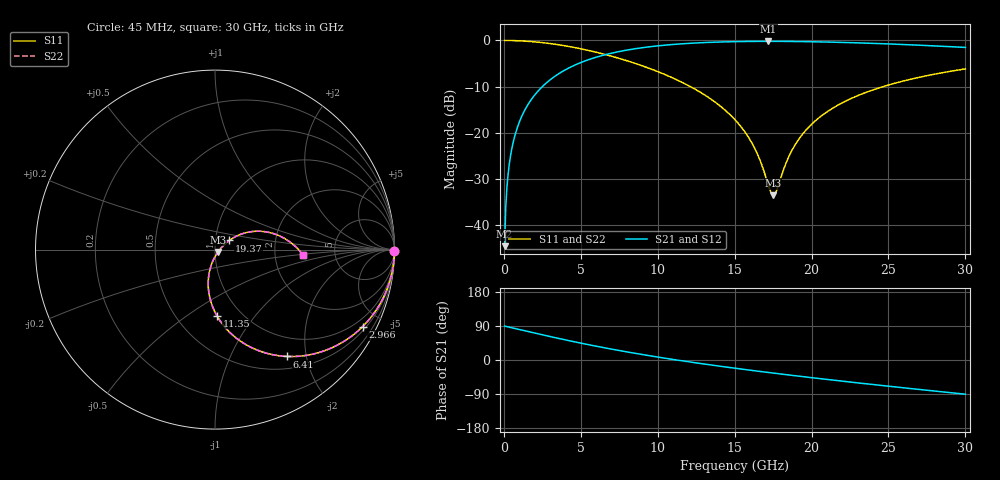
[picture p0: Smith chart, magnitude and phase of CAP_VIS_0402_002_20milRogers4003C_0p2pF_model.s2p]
! S-parameter model data by Modelithics Inc.  support@modelithics.com  813-866-6335  Tampa FL USA
! S-Parameter data specifications:
! Substrate: 20-mil Rogers 4003C, substrate thickness, H=0.508mm, Dielectric constant, Er=3.75
! PCB Mounting Pad Footprint: Pad width, PadW=0.50mm , Pad length, PadL=0.50mm , Pad gap, PadG (edge-to-edge)=0.40mm , Reference planes=1.4mm apart
! Created Wed Nov 18 12:41:56 2015
# hz S ma R 50
! 2 Port Network Data from SP1.SP block
! freq  magS11  angS11  magS21  angS21  magS12  angS12  magS22  angS22
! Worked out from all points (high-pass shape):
!   401 points, 45 MHz to 30 GHz, reference 50 ohm
!   highest |S21| = -0.19 dB at 17.19 GHz (marker M1); lowest = -44.5 dB at 45 MHz (marker M2)
!   |S21| within 3 dB of the highest: 6.465 GHz to end of sweep
!   lowest |S11| = -33.5 dB at 17.49 GHz (marker M3), VSWR 1.04, Z = 51.7 - j1.36 ohm
!   |S11| at or under -10 dB: 12.13 GHz to 24.65 GHz (12.52 GHz wide, 68.1 % of centre)
!   |S22| runs from -33.5 to 0.0 dB; largest |S21 - S12| = 0
!   S11 on the Smith chart (normalised r, x): 45 MHz: open; 2.966 GHz: 0.65, -3.97; 6.41 GHz: 0.68, -1.66; 11.35 GHz: 0.78, -0.66; 19.37 GHz: 1.17, +0.12; 30 GHz: 2.92, -0.24
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4.5e7  1 -0.4  0.00593 89.5  0.00593 89.5  1 -0.4
3.4455e8  0.9989 -3.3  0.04525 86.6  0.04525 86.6  0.9989 -3.3
5.692125e8  0.9971 -5.4  0.07461 84.5  0.07461 84.5  0.9971 -5.4
7.93875e8  0.9944 -7.5  0.1038 82.4  0.1038 82.4  0.9944 -7.5
1.617638e9  0.9774 -15.3  0.2091 74.6  0.2091 74.6  0.9774 -15.3
2.965612e9  0.9273 -27.6  0.3707 62.2  0.3707 62.2  0.9273 -27.6
5.062462e9  0.8084 -45.6  0.5821 44.0  0.5821 44.0  0.8084 -45.6
6.410438e9  0.7167 -56.2  0.6888 33.2  0.6888 33.2  0.7167 -56.2
1.007992e10  0.4547 -81.1  0.8769 7.2  0.8769 7.2  0.4547 -81.1
1.135301e10  0.3675 -88.5  0.9147 -0.8  0.9147 -0.8  0.3675 -88.5
1.344986e10  0.2323 -98.8  0.955 -13.1  0.955 -13.1  0.2323 -98.8
1.50225e10  0.1385 -103.9  0.9711 -21.7  0.9711 -21.7  0.1385 -103.9
1.629559e10  0.06843 -101.3  0.9773 -28.4  0.9773 -28.4  0.06843 -101.3
1.719424e10  0.02698 -72.4  0.9784 -33.0  0.9784 -33.0  0.02698 -72.4
1.749379e10  0.02115 -38.4  0.9783 -34.5  0.9783 -34.5  0.02115 -38.4
1.771845e10  0.0236 -10.1  0.9781 -35.6  0.9781 -35.6  0.0236 -10.1
1.86171e10  0.05967 28.3  0.9758 -40.0  0.9758 -40.0  0.05967 28.3
1.936598e10  0.09454 32.6  0.9725 -43.6  0.9725 -43.6  0.09454 32.6
2.003996e10  0.1256 32.6  0.9686 -46.8  0.9686 -46.8  0.1256 32.6
2.213681e10  0.2172 27.0  0.9511 -56.5  0.9511 -56.5  0.2172 27.0
2.505742e10  0.3314 16.0  0.9165 -69.4  0.9165 -69.4  0.3314 16.0
3e10  0.4924 -3.7  0.8403 -90.3  0.8403 -90.3  0.4924 -3.7
